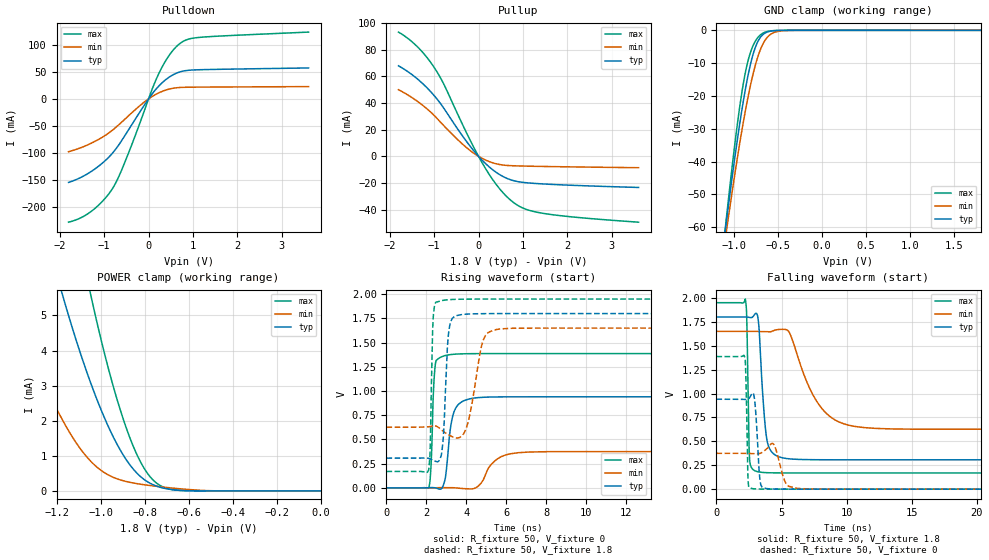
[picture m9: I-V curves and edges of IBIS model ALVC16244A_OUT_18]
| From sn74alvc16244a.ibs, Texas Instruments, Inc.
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[Model]   ALVC16244A_OUT_18
Model_type  3-state
Enable   Active-Low
Vref =   0
Rref =   1k
Cref =   30p
Vmeas =   0.9
| variable   typ   min   max
C_comp   2.62pF   2.27pF   2.76pF
| C_pullup   3.58pF   3.11pF   4.18pF
| C_pulldown   5.17pF   3.66pF   6.71pF
| C_tri-state   2.62pF   2.27pF   2.76pF
[Temperature Range]   40   100   -40
| Ambient temperature   25   85   -40
[Voltage range]   1.8   1.65   1.95
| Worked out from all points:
|   slope of the pulldown table from 0 to 0.27 V, typ, clamps not added: 10 ohm
|   slope of the pullup table from 0 to 0.27 V, typ, clamps not added: 30.8 ohm
|   GND clamp passes 1 mA (typ) near -0.66 V on its own axis
|   POWER clamp passes 1 mA (typ) near -0.89 V on its own axis
|   rising waveform, R_fixture 50, V_fixture 0: 20-80 % time 332ps typ, 742ps min, 139ps max; typ from 0 V to 0.94 V
|   falling waveform, R_fixture 50, V_fixture 1.8: 20-80 % time 440ps typ, 2.07ns min, 137ps max; typ from 1.8 V to 0.307 V
|   rising waveform, R_fixture 50, V_fixture 1.8: 20-80 % time 198ps typ, 494ps min, 106ps max; typ from 0.307 V to 1.8 V
|   falling waveform, R_fixture 50, V_fixture 0: 20-80 % time 237ps typ, 485ps min, 121ps max; typ from 0.94 V to 0 V
[GND Clamp]
| ALVC16244A_OUT_18
|   Voltage   I(typ)   I(min)   I(max)
-1.8V     -231.4mA   -215.3mA   -257.8mA
-1.1V     -61.03mA   -63.82mA   -60.43mA
-1.085V   -57.84mA   -60.98mA   -56.71mA
-1.07V    -54.69mA   -58.15mA   -53.03mA
-960mV    -32.92mA   -38.51mA   -28.12mA
-875mV    -18.55mA   -25.08mA   -13.37mA
-830mV    -12.34mA   -18.85mA   -8.18mA
-775mV    -6.546mA   -12.35mA   -4.159mA
-675mV    -1.374mA   -4.329mA   -903.1uA
-575mV    -204.7uA   -1.042mA   -147.9uA
-425mV    -10.46uA   -85.14uA   -10.28uA
1.8V      2.304nA    59.8nA     11.39nA
[POWER Clamp]
| ALVC16244A_OUT_18
|   Voltage   I(typ)   I(min)   I(max)
-1.8V     25.11mA    14.19mA    39.93mA
-1.415V   11.83mA    5.639mA    19.65mA
-1.18V    5.742mA    2.103mA    9.959mA
-1.165V   5.414mA    1.93mA     9.427mA
-1.045V   3.081mA    848uA      5.599mA
-960mV    1.772mA    439.6uA    3.385mA
-895mV    1.004mA    286.9uA    2.013mA
-840mV    542.1uA    213.8uA    1.108mA
-790mV    274.5uA    166.5uA    530uA
-735mV    115uA      123.6uA    176.7uA
-610mV    7.213uA    44.53uA    5.785uA
-16.28fV  2.304nA    59.66nA    11.28nA
[Pulldown]
| ALVC16244A_OUT_18
|   Voltage   I(typ)   I(min)   I(max)
-1.8V     -154.3mA   -97.53mA   -227.7mA
-1.275V   -133.3mA   -81.3mA    -206.8mA
-1.01V    -116.6mA   -69.28mA   -186.7mA
-805mV    -99.61mA   -57.35mA   -164.8mA
-505mV    -64.22mA   -35.41mA   -111.3mA
-20mV     -2.398mA   -1.172mA   -4.654mA
210mV     21.85mA    10.32mA    43.05mA
450mV     39.36mA    17.78mA    78.77mA
695mV     49.56mA    20.99mA    101.6mA
880mV     52.63mA    21.52mA    109.8mA
1.15V     53.84mA    21.74mA    113.6mA
3.6V      57.13mA    22.68mA    123.4mA
[Pullup]
| ALVC16244A_OUT_18
|   Voltage   I(typ)   I(min)   I(max)
-1.8V     67.82mA    49.93mA    93.11mA
-1.38V    58.14mA    41.32mA    82.29mA
-1.19V    52.37mA    36.44mA    75.34mA
-1.01V    45.98mA    31mA       67.22mA
-780mV    36mA       22.96mA    54.02mA
-340mV    14.33mA    8.546mA    22.47mA
105mV     -3.708mA   -1.929mA   -6.218mA
440mV     -12.97mA   -5.934mA   -22.89mA
760mV     -17.99mA   -7.06mA    -33.91mA
1.05V     -19.72mA   -7.341mA   -39.49mA
1.46V     -20.73mA   -7.61mA    -42.78mA
3.6V      -23.36mA   -8.546mA   -49.39mA
[Ramp]
| ALVC16244A_OUT_18
| variable   typ   min   max
dV/dt_r   0.57/3.46E-10   0.23/7.54E-10   0.83/1.48E-10
dV/dt_f   0.92/4.53E-10   0.63/2.08E-09   1.09/1.50E-10
R_load = 50
[Rising Waveform]
| ALVC16244A_OUT_18
R_fixture =   50
C_fixture =   0
L_fixture =   0
V_fixture =   0
V_fixture_min = 0
V_fixture_max = 0
|   Time   V(typ)   V(min)   V(max)
0s        258.6pV    441.2pV    154.1pV
2.11ns    1.742mV    -205.1uV   -3.916mV
2.225ns   2.789mV    -388.7uV   211.6mV
2.455ns   -203.2uV   629.7uV    1.288V
2.915ns   73.96mV    2.002mV    1.365V
3.165ns   557.8mV    1.627mV    1.375V
3.61ns    863.6mV    -3.172mV   1.383V
4.9ns     935.9mV    106.9mV    1.387V
7.125ns   940.3mV    369.9mV    1.387V
50ns      940.4mV    374.9mV    1.387V
[Falling Waveform]
| ALVC16244A_OUT_18
R_fixture =   50
C_fixture =   0
L_fixture =   0
V_fixture =   1.8
V_fixture_min = 1.65
V_fixture_max = 1.95
|   Time   V(typ)   V(min)   V(max)
0s        1.8V       1.65V      1.95V
2.22ns    1.8V       1.65V      1.983V
2.325ns   1.8V       1.65V      1.785V
2.545ns   1.796V     1.65V      313.3mV
3.125ns   1.826V     1.65V      184mV
3.87ns    519.7mV    1.647V     172.6mV
5.015ns   329.5mV    1.672V     169.8mV
7.95ns    307.7mV    868.5mV    169.4mV
10.58ns   307.1mV    657mV      169.4mV
50ns      307mV      625.8mV    169.4mV
[Rising Waveform]
| ALVC16244A_OUT_18
R_fixture =   50
C_fixture =   0
L_fixture =   0
V_fixture =   1.8
V_fixture_min = 1.65
V_fixture_max = 1.95
|   Time   V(typ)   V(min)   V(max)
0s        307mV      625.9mV    169.4mV
2.11ns    304.6mV    631.1mV    182.9mV
2.18ns    299.4mV    632.7mV    363.5mV
2.35ns    282.5mV    638.9mV    1.788V
2.835ns   495.5mV    584.7mV    1.937V
3.125ns   1.624V     545.4mV    1.944V
3.765ns   1.79V      534.4mV    1.949V
4.835ns   1.799V     1.519V     1.95V
5.705ns   1.8V       1.642V     1.95V
50ns      1.8V       1.65V      1.95V
[Falling Waveform]
| ALVC16244A_OUT_18
R_fixture =   50
C_fixture =   0
L_fixture =   0
V_fixture =   0
V_fixture_min = 0
V_fixture_max = 0
|   Time   V(typ)   V(min)   V(max)
0s        940.4mV    374.9mV    1.387V
2.17ns    938.6mV    374.3mV    1.379V
2.265ns   938.3mV    374mV      1.141V
2.43ns    941.4mV    373.4mV    94.42mV
2.725ns   999.9mV    372mV      6.735mV
2.965ns   887.4mV    370.7mV    3.003mV
3.365ns   74mV       375.4mV    1.081mV
3.81ns    7.186mV    416.1mV    386.3uV
6.475ns   67.13uV    5.436mV    2.194uV
50ns      1.8uV      -11.03nV   2.393nV
